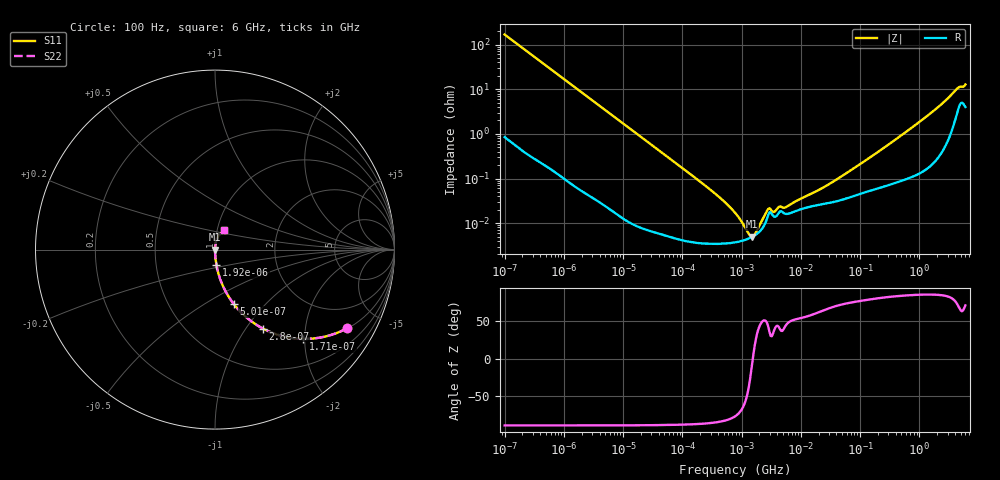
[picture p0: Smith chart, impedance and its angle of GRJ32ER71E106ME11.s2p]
!Murata Part Number: GRJ32ER71E106ME11
!These Parameters are Measured in Series Mode Connection
!Data Generated on Jun 19, 2026
!  o--ll--o
!Port1  Port2
!  o------o
!Operation Temp=25[degC], DC Bias Voltage=0[V]
!Freq. Start=100[Hz] Stop=6[GHz] 401[Steps]
# Hz S RI R 50
!Freq.(Hz) S11(Real) S11(Imag) S21(Real) S21(Imag) S12(Real) S12(Imag) S22(Real) S22(Imag)
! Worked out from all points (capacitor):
!   401 points, 100 Hz to 6 GHz, reference 50 ohm
!   read as one part in series: C = 9.46 uF near 109 Hz
!   lowest |Z| = 4.97 mohm at 1.516 MHz (marker M1)
!   series resonance near 1.549 MHz, so ESL is about 1.1 nH
!   S11 on the Smith chart (normalised r, x): 100 Hz: 1.02, -3.36; 171 Hz: 1.01, -1.97; 280 Hz: 1.01, -1.20; 501 Hz: 1.00, -0.67; 1.92 kHz: 1.00, -0.18; 6 GHz: 1.08, +0.24
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100  0.7375 -0.4375  0.2625 0.4375  0.2625 0.4375  0.7375 -0.4375
171  0.4919 -0.4975  0.5081 0.4975  0.5081 0.4975  0.4919 -0.4975
280  0.2671 -0.4399  0.7329 0.4399  0.7329 0.4399  0.2671 -0.4399
501  0.1033 -0.3016  0.8967 0.3016  0.8967 0.3016  0.1033 -0.3016
1920  0.00828 -0.0876  0.9917 0.0876  0.9917 0.0876  0.00828 -0.0876
2008  0.00761 -0.0839  0.9924 0.0839  0.9924 0.0839  0.00761 -0.0839
40335  7.62e-05 -0.00425  0.9999 0.00425  0.9999 0.00425  7.62e-05 -0.00425
330837  3.46e-05 -0.000499  1 0.000499  1 0.000499  3.46e-05 -0.000499
774597  3.71e-05 -0.000168  1 0.000168  1 0.000168  3.71e-05 -0.000168
1059725  4.07e-05 -8.73e-05  1 8.73e-05  1 8.73e-05  4.07e-05 -8.73e-05
1516199  4.95e-05 -4.8e-06  1 4.8e-06  1 4.8e-06  4.95e-05 -4.8e-06
2074311  6.75e-05 7.02e-05  0.9999 -7.02e-05  0.9999 -7.02e-05  6.75e-05 7.02e-05
2837864  0.000155 0.000142  0.9998 -0.000142  0.9998 -0.000142  0.000155 0.000142
3549919  0.00014 0.000111  0.9999 -0.000111  0.9999 -0.000111  0.00014 0.000111
4440638  0.000182 0.000152  0.9998 -0.000152  0.9998 -0.000152  0.000182 0.000152
5554849  0.000161 0.000159  0.9998 -0.000159  0.9998 -0.000159  0.000161 0.000159
1.555665e7  0.00024 0.0004  0.9998 -0.0004  0.9998 -0.0004  0.00024 0.0004
4.35672e7  0.000319 0.000966  0.9997 -0.000966  0.9997 -0.000966  0.000319 0.000966
3.124326e8  0.000753 0.00589  0.9992 -0.00589  0.9992 -0.00589  0.000753 0.00589
1.637704e9  0.00297 0.0304  0.997 -0.0304  0.997 -0.0304  0.00297 0.0304
4.385646e9  0.0383 0.0928  0.9617 -0.0928  0.9617 -0.0928  0.0383 0.0928
6e9  0.0512 0.1102  0.9488 -0.1102  0.9488 -0.1102  0.0512 0.1102
